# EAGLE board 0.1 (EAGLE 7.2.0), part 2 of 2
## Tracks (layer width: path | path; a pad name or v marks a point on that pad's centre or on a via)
3.12V-FIXED  (2 unrouted)
4X-TEMPSWITCHES-COMBINED  (3 unrouted)
+5VDC  (17 unrouted)
+5VDC-IN  (2 unrouted)
+15VDC  (67 unrouted)
+15VDC-IN  (2 unrouted)
+15VDC-PSU  (4 unrouted)
+33VDC-IN  (1 unrouted)
-15VDC  (22 unrouted)
-15VDC-IN  (2 unrouted)
??12  (1 unrouted)
AC-BAL-VOLTAGE-1  (2 unrouted)
AC-BAL-VOLTAGE-2  (1 unrouted)
AC-BAL-VOLTAGE-INVERTED  (3 unrouted)
AC-BAL-VOLTAGE-INVERTED-TRIANGLE-TRIGGER-VOLTS  (2 unrouted)
AC-BALANCE/0V=20%EP  (1 unrouted)
AC-BALANCED-AC-FREQ-PULSES-1  (2 unrouted)
AC-BALANCED-AC-FREQ-PULSES-2  (1 unrouted)
AC-BALANCED-AC-FREQ-PULSES-3  (3 unrouted)
AC-BALANCED-AC-FREQ-PULSES-4  (4 unrouted)
AC-FREQ-TRIANGLE-1  (5 unrouted)
AC-FREQ-TRIANGLE-2  (2 unrouted)
AC-FREQ-VADJ-3  (1 unrouted)
AC-FREQ-VOLTAGE-2  (4 unrouted)
AC-FREQ-VOLTAGE-ADJUSTED  (3 unrouted)
AC-FREQ-VOLTAGE-BUFFERED  (2 unrouted)
AC-FREQ-VOLTAGE-BUFFERED-ADJ-1  (1 unrouted)
AC-FREQ-VOLTAGE-BUFFERED-ADJ-2  (3 unrouted)
AC-FREQ-VOLTAGE-IN  (4 unrouted)
AC-FREQ-VOLTS/3.12V-FIXED  (3 unrouted)
AC-FREQ-VOLTS/3.12V-FIXED-2  (2 unrouted)
AC-FREQ/0V=50HZ  (1 unrouted)
AC-NEG-RAMP-CURRENT  (1 unrouted)
AC-POS-RAMP-CURRENT  (1 unrouted)
AC-SQUAREWAVE-(FROM-AC-TRIANGLE)=>TRIANGLE-INTEGRATOR-BIAS-SWITCH&MINUS-LED  (6 unrouted)
AC/DC-AC=15V  (3 unrouted)
ALL-TEMPSWITCHES-COMBINED  (4 unrouted)
CHOPPER-AC-FREQ  (3 unrouted)
D6-D7-SWITCH-ENABLE  (3 unrouted)
D6-D7-SWITCH-ENABLE-1  (1 unrouted)
D6-D7-SWITCH-ENABLE-2  (1 unrouted)
D8-SWITCH-ENABLE-(FIXED/VARIABLE-AC-FREQ)  (6 unrouted)
D8-SWITCH-ENABLE-(FIXED/VARIABLE-AC-FREQ)-FROM-X1/2&X3/2  (2 unrouted)
GND  (197 unrouted)
I-PULS  (1 unrouted)
INP-1/1-AC-SWITCH-DELAY?  (5 unrouted)
INP-1/7-  (4 unrouted)
INP-4/X-TEMP-SWITCHES  (2 unrouted)
INP-5/X-  (3 unrouted)
INP-6/X-  (4 unrouted)
INP-7/X-  (3 unrouted)
INP-8/X-  (2 unrouted)
INP-11/X-  (4 unrouted)
INP-X/2-N5-TEMP-SENSOR-(0=>GOOD)  (7 unrouted)
INP-X/3-FIXED/VARIABLE-AC-FREQ  (3 unrouted)
INP-X/5-  (1 unrouted)
INP-X/6-PLUS-MINUS-NOT-D6-D7-SWITCH-ENABLE-1  (3 unrouted)
INP-X/15-FROM-OUTP-X/22  (2 unrouted)
INP-X/23-FROM-OUTP-X/15  (2 unrouted)
INV-AC-FREQ-VOLTS/-3.12V-FIXED  (2 unrouted)
N5-NEG-INP  (3 unrouted)
N5-POS-INP  (1 unrouted)
N5-TEMP-OUT  (2 unrouted)
N5-TEMP-OUT-2  (2 unrouted)
N5-TEMP-OUT-3  (2 unrouted)
N9-8-FIXED-VOLTAGE-LEVEL  (3 unrouted)
N10-P4/+2.411VDC-FIXED  (3 unrouted)
N10-P9-FIXED-VOLTAGE-AC-SWITCH-DELAY?  (2 unrouted)
N10-P11-FIXED-VOLTAGE  (2 unrouted)
N12-P2-TO-GND  (1 unrouted)
N12-P5-TO-GND  (1 unrouted)
N12-P9-TO-GND  (1 unrouted)
N12-P13-FIXED-VOLTAGE  (2 unrouted)
N$1  (1 unrouted)
N$2  (1 unrouted)
N$4  (1 unrouted)
N$5  (2 unrouted)
N$6  (1 unrouted)
N$7  (7 unrouted)
N$8  (2 unrouted)
N$9  (2 unrouted)
N$12  (5 unrouted)
N$13  (2 unrouted)
N$14  (5 unrouted)
N$17  (6 unrouted)
N$18  (3 unrouted)
N$19  (1 unrouted)
N$20  (1 unrouted)
N$21  (2 unrouted)
N$22  (1 unrouted)
N$23  (1 unrouted)
N$24  (1 unrouted)
N$25  (2 unrouted)
N$26  (1 unrouted)
N$27  (2 unrouted)
N$28  (3 unrouted)
N$29  (3 unrouted)
N$30  (4 unrouted)
N$33  (4 unrouted)
N$34  (1 unrouted)
N$35  (1 unrouted)
N$36  (1 unrouted)
N$37  (2 unrouted)
N$38  (4 unrouted)
N$39  (2 unrouted)
N$45  (3 unrouted)
N$50  (4 unrouted)
N$51  (1 unrouted)
N$52  (2 unrouted)
N$53  (1 unrouted)
N$54  (1 unrouted)
N$55  (4 unrouted)
N$56  (4 unrouted)
N$57  (3 unrouted)
N$58  (2 unrouted)
N$59  (4 unrouted)
N$66  (5 unrouted)
N$67  (1 unrouted)
N$70  (3 unrouted)
N$72  (1 unrouted)
N$74  (1 unrouted)
N$75  (1 unrouted)
N$78  (1 unrouted)
N$79  (1 unrouted)
N$81  (1 unrouted)
N$84  (3 unrouted)
N$86  (1 unrouted)
N$89  (4 unrouted)
N$90  (1 unrouted)
N$91  (4 unrouted)
N$92  (2 unrouted)
N$93  (1 unrouted)
N$94  (2 unrouted)
N$95  (1 unrouted)
N$96  (3 unrouted)
N$97  (1 unrouted)
N$98  (1 unrouted)
N$100  (1 unrouted)
N$101  (1 unrouted)
N$102  (1 unrouted)
N$103  (1 unrouted)
N$104  (1 unrouted)
N$105  (1 unrouted)
N$106  (2 unrouted)
N$111  (1 unrouted)
N$114  (1 unrouted)
N$116  (1 unrouted)
N$117  (1 unrouted)
N$122  (2 unrouted)
N$127  (2 unrouted)
N$130  (1 unrouted)
N$133  (1 unrouted)
N$134  (1 unrouted)
N$135  (1 unrouted)
N$137  (3 unrouted)
N$139  (1 unrouted)
N$140  (1 unrouted)
N$141  (1 unrouted)
N$142  (2 unrouted)
N$144  (2 unrouted)
N$145  (1 unrouted)
N$146  (2 unrouted)
N$147  (1 unrouted)
N$148  (1 unrouted)
N$149  (2 unrouted)
N$151  (2 unrouted)
N$152  (1 unrouted)
N$153  (1 unrouted)
N$154  (1 unrouted)
N$155  (1 unrouted)
N$156  (2 unrouted)
N$157  (2 unrouted)
N$158  (2 unrouted)
N$160  (1 unrouted)
N$161  (1 unrouted)
N$165  (2 unrouted)
N$166  (1 unrouted)
N$167  (1 unrouted)
N$168  (2 unrouted)
N$171  (4 unrouted)
N$177  (3 unrouted)
N$182  (1 unrouted)
N$184  (1 unrouted)
N$187  (1 unrouted)
N$189  (1 unrouted)
N$190  (1 unrouted)
N$192  (1 unrouted)
N$198  (2 unrouted)
N$199  (4 unrouted)
N$203  (1 unrouted)
N$204  (3 unrouted)
N$205  (1 unrouted)
N$206  (2 unrouted)
N$207  (4 unrouted)
N$208  (3 unrouted)
N$209  (1 unrouted)
N$210  (1 unrouted)
N$211  (1 unrouted)
N$212  (1 unrouted)
N$213  (2 unrouted)
N$214  (3 unrouted)
N$215  (1 unrouted)
N$218  (4 unrouted)
N$219  (2 unrouted)
N$221  (5 unrouted)
N$224  (2 unrouted)
N$225  (2 unrouted)
N$226  (1 unrouted)
N$227  (2 unrouted)
N$228  (2 unrouted)
N$229  (2 unrouted)
N$230  (3 unrouted)
N$231  (2 unrouted)
N$232  (1 unrouted)
N$233  (1 unrouted)
N$234  (1 unrouted)
N$235  (4 unrouted)
N$236  (2 unrouted)
N$237  (1 unrouted)
N$238  (2 unrouted)
N$239  (1 unrouted)
N$240  (2 unrouted)
N$241  (2 unrouted)
N$242  (2 unrouted)
N$243  (2 unrouted)
N$244  (4 unrouted)
N$245  (2 unrouted)
N$246  (1 unrouted)
N$247  (1 unrouted)
N$250  (4 unrouted)
N$252  (1 unrouted)
N$253  (1 unrouted)
N$254  (2 unrouted)
N$255  (1 unrouted)
N$256  (3 unrouted)
N$257  (1 unrouted)
N$258  (2 unrouted)
N$259  (1 unrouted)
N$260  (1 unrouted)
N$261  (1 unrouted)
N$262  (1 unrouted)
N$264  (1 unrouted)
N$265  (1 unrouted)
N$268  (1 unrouted)
N$270  (3 unrouted)
N$273  (1 unrouted)
N$274  (4 unrouted)
N$275  (1 unrouted)
N$277  (1 unrouted)
N$278  (1 unrouted)
N$280  (4 unrouted)
N$281  (1 unrouted)
N$282  (1 unrouted)
N$283  (1 unrouted)
N$284  (1 unrouted)
N$285  (1 unrouted)
N$286  (1 unrouted)
N$288  (1 unrouted)
N$289  (2 unrouted)
N$291  (2 unrouted)
N$292  (2 unrouted)
N$295  (3 unrouted)
N$296  (1 unrouted)
N$297  (1 unrouted)
N$298  (3 unrouted)
N$299  (1 unrouted)
N$300  (1 unrouted)
N$302  (5 unrouted)
N$303  (1 unrouted)
N$304  (5 unrouted)
N$305  (1 unrouted)
N$306  (3 unrouted)
N$307  (3 unrouted)
N$308  (2 unrouted)
N$309  (1 unrouted)
N$310  (1 unrouted)
N$311  (1 unrouted)
N$312  (2 unrouted)
N$313  (1 unrouted)
N$314  (1 unrouted)
N$316  (1 unrouted)
N$317  (6 unrouted)
N$318  (2 unrouted)
N$320  (4 unrouted)
N$323  (1 unrouted)
N$325  (1 unrouted)
N$326  (1 unrouted)
N$334  (2 unrouted)
N$335  (1 unrouted)
N$336  (1 unrouted)
N$337  (1 unrouted)
N$338  (1 unrouted)
N$340  (1 unrouted)
N$341  (1 unrouted)
N$342  (3 unrouted)
N$344  (2 unrouted)
N$346  (1 unrouted)
N$347  (2 unrouted)
N$348  (1 unrouted)
N$349  (1 unrouted)
N$350  (1 unrouted)
N$354  (1 unrouted)
N$356  (2 unrouted)
N$358  (1 unrouted)
N$360  (2 unrouted)
N$361  (2 unrouted)
N$363  (2 unrouted)
N$364  (2 unrouted)
N$365  (1 unrouted)
N$366  (1 unrouted)
N$367  (1 unrouted)
N$368  (4 unrouted)
N$369  (3 unrouted)
N$370  (2 unrouted)
N$371  (2 unrouted)
N$372  (3 unrouted)
N$373  (4 unrouted)
N$374  (2 unrouted)
N$375  (1 unrouted)
N$376  (2 unrouted)
N$377  (2 unrouted)
N$378  (1 unrouted)
N$379  (3 unrouted)
N$382  (2 unrouted)
N$385  (2 unrouted)
NEG-2.5V-REFERENCE-VOLTAGE  (2 unrouted)
NOT-NOT-D6-D7-SWITCH-ENABLE-1  (3 unrouted)
OUTP-12/X-TEMP-LED  (2 unrouted)
OUTP-13/X-SEKUE-LED  (2 unrouted)
OUTP-14/X-UNUSED?  (4 unrouted)
OUTP-15/X-PRUN-LED  (3 unrouted)
OUTP-16/X-UNUSED?  (3 unrouted)
OUTP-17/X-STOER-LED  (2 unrouted)
OUTP-18/X-D10-VARIABLE/FIXED-AC-BAL/IGRO-LED  (4 unrouted)
OUTP-19/INP-8  (3 unrouted)
OUTP-X/15-TO-INP-X/23  (1 unrouted)
OUTP-X/16-POLARITY  (2 unrouted)
OUTP-X/17-OUTP-X/18-X11-POS-OPC-X10-NEG-OPC  (3 unrouted)
OUTP-X/18-X10-POS-OPC-X11-NEG-OPC  (4 unrouted)
OUTP-X/19-UNUSED?-ALWAYS=1  (2 unrouted)
OUTP-X/20  (2 unrouted)
OUTP-X/21-D14-ENABLE-LOGIC  (1 unrouted)
OUTP-X/22-TO-INP-X/14  (1 unrouted)
P8-P1=>+15V  (1 unrouted)
P10-P1=>GND  (1 unrouted)
PLUS/MINUS-1  (1 unrouted)
PLUS/MINUS-2  (3 unrouted)
POLAR  (3 unrouted)
REF-VNEG  (1 unrouted)
SEKUE-LED-DRIVE  (1 unrouted)
STOERUNG-LED  (1 unrouted)
STOERUNG-LED-DRIVE-OUT  (3 unrouted)
TO-GND-R-1  (1 unrouted)
TO-GND-R-192  (1 unrouted)
TO-INP-11/X-  (1 unrouted)
TRIANGLE-INPUT=>SQUAREWAVE  (3 unrouted)
TRIANGLE-INTEGRATOR-VARIABLE-BIAS-CURRENT-(AC-FREQ)  (3 unrouted)
X1-TEMPSWITCH-1  (2 unrouted)
X1-TEMPSWITCH-2  (2 unrouted)
X10-4-OPTOCOUPL-POS  (1 unrouted)
X10-5-OPTOCOUPL-NEG  (1 unrouted)
X11-4-OPTOCOUPL-POS  (1 unrouted)
X11-5-OPTOCOUPL-NEG  (1 unrouted)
